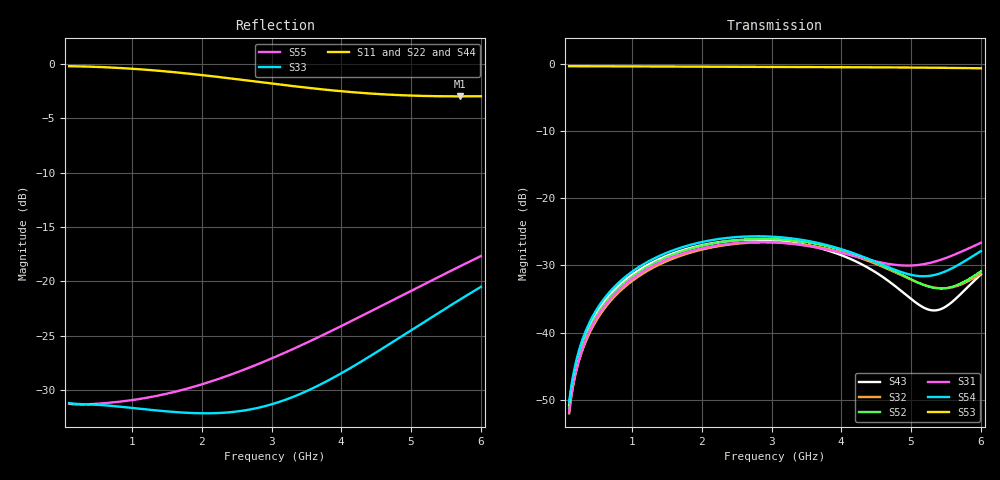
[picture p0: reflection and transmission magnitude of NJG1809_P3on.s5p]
! Port1:P1  Port2:P2  Port3:P3  Port4:P4  Port5:PC
# hz S ma R 50
! 5 Port Network Data from SP1.SP block
! freq  magS11  angS11  magS12  angS12  magS13  angS13  magS14  angS14
!  magS15  angS15
!  magS21  angS21  magS22  angS22  magS23  angS23
!  magS24  angS24  magS25  angS25
!  magS31  angS31  magS32  angS32
!  magS33  angS33  magS34  angS34  magS35  angS35
!  magS41  angS41
!  magS42  angS42  magS43  angS43  magS44  angS44  magS45  angS45
!  magS51  angS51  magS52  angS52  magS53  angS53  magS54  angS54
!  magS55  angS55
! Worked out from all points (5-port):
!   591 points, 100 MHz to 6 GHz, reference 50 ohm
!   strongest paths, dB at 100 MHz, 1.57 GHz, 3.05 GHz, 4.53 GHz, 6 GHz:
!     S53: -0.4, -0.4, -0.5, -0.5, -0.7
!     S54: -50.4, -27.8, -25.8, -29.6, -27.9
!     S31: -51.9, -28.8, -26.6, -29.5, -26.6
!     S52: -51.2, -28.5, -26.1, -29.7, -30.9
!     S32: -52.0, -29.1, -26.6, -29.9, -31.2
!     S43: -50.8, -28.3, -26.3, -31.3, -31.3
!   lowest |S11| = -3.0 dB at 5.7 GHz (marker M1), VSWR 5.92, Z = 10.7 + j25.4 ohm
!   |S11| at or under -10 dB: nowhere
